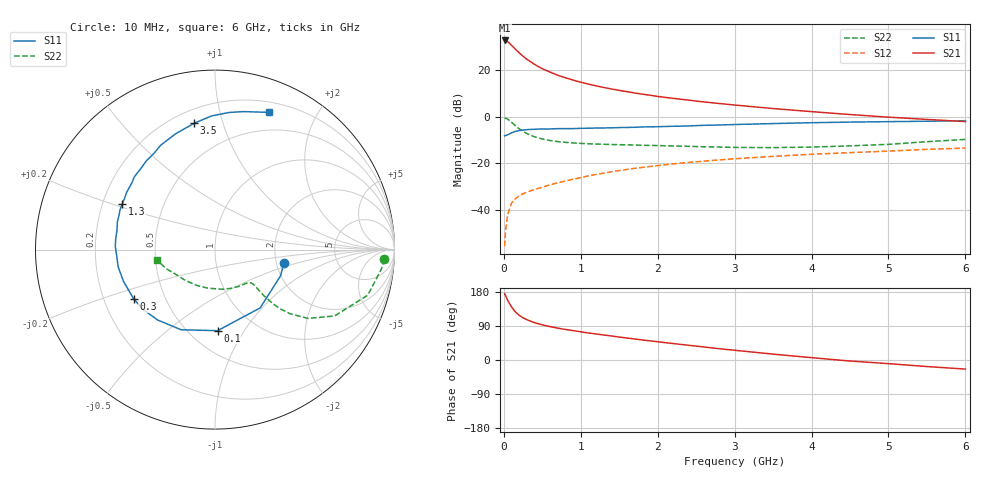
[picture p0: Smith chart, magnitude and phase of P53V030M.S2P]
! SIEMENS Small Signal Semiconductors
! BFP183
! Si NPN RF Bipolar Junction Transistor in SOT143
! VCE = 3 V  IC = 30 mA
! Common Emitter S-Parameters:  March  1996
# GHz  S  MA  R  50
!  f  S11  S21  S12  S22
! GHz  MAG  ANG  MAG  ANG  MAG  ANG  MAG  ANG
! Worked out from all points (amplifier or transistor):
!   36 points, 10 MHz to 6 GHz, reference 50 ohm
!   highest |S21| = 32.6 dB at 10 MHz (marker M1)
!   |S21| within 3 dB of that: start of sweep to 128.5 MHz
!   unconditionally stable (mu >= 1): 620.6 MHz to 5.685 GHz
!   at 250 MHz: K = 0.61, MSG = 29.4 dB, |S12| = -33.0 dB
!   at 1.4 GHz: K = 1.18, MAG = 15.1 dB, |S12| = -23.6 dB
!   at 6 GHz: K = 0.96, MSG = 5.7 dB, |S12| = -13.4 dB
!   S11 on the Smith chart (normalised r, x): 10 MHz: 2.20, -0.39; 100 MHz: 0.68, -0.77; 300 MHz: 0.33, -0.25; 1.3 GHz: 0.28, +0.21; 3.5 GHz: 0.28, +0.81; 6 GHz: 0.30, +1.43
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0.01  0.3915 -11.2  42.87 175.2  0.0017 86.2  0.9452 -3.2
0.02  0.3933 -21.8  42.54 170.9  0.0033 74.6  0.9331 -6.7
0.05  0.4109 -52.2  40.4 157.5  0.0082 76.2  0.8884 -16.6
0.1  0.452 -88.2  33.82 139.9  0.0141 61.9  0.7623 -29.0
0.15  0.4848 -112.9  27.97 127.0  0.0177 56.2  0.6447 -36.5
0.2  0.5058 -129.2  23.28 117.9  0.0202 53.2  0.5526 -40.4
0.25  0.521 -140.0  19.62 111.3  0.0225 51.8  0.4857 -42.4
0.3  0.5299 -148.9  16.95 106.3  0.0244 51.3  0.4357 -43.1
0.4  0.5397 -160.9  13.15 98.4  0.0277 52.2  0.3718 -43.3
0.5  0.5481 -169.9  10.65 92.8  0.031 52.9  0.3335 -42.8
0.6  0.5485 -176.2  9.029 88.1  0.035 54.2  0.3101 -42.4
0.7  0.5561 178.0  7.72 84.1  0.0385 56.1  0.294 -42.2
0.8  0.5566 173.0  6.827 80.6  0.0421 56.8  0.2833 -42.2
1.1  0.5675 160.8  4.995 71.3  0.0542 57.5  0.2638 -44.2
1.3  0.5755 154.0  4.215 65.9  0.0621 56.9  0.2575 -46.6
1.7  0.5948 140.9  3.221 55.5  0.0785 55.2  0.248 -53.2
2.2  0.6252 127.7  2.474 43.4  0.0978 51.3  0.2365 -63.5
2.8  0.6658 113.4  1.92 29.8  0.1192 45.7  0.2248 -79.3
3.5  0.7138 99.3  1.496 15.5  0.1418 39.3  0.2185 -100.8
4.5  0.768 84.1  1.114 -2.7  0.1706 29.7  0.2381 -133.7
5.5  0.8008 73.2  0.876 -17.3  0.2004 21.6  0.2923 -158.8
6  0.8223 68.4  0.788 -24.0  0.2133 16.9  0.3273 -169.5
